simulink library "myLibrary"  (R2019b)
settings: Solver=VariableStepAuto  StartTime=0.0  StopTime=10.0  RelTol=1e-3
undefined symbols (not defined in the file or in its folder): batt_delay, Calculation, cap_1ph, cap_3ph, Complex, Current, Dynamic, EV, ev_charger, EV_ID, ev_num, gcbh, Iabc, Load, max_charge_1ph, max_charge_3ph, max_disch_1ph, max_disch_3ph, MV_LV_transf, myLibrary, phase, Phase, Phasor, rated_1ph, rated_3ph, Single, SoC_init, SPDL, sps_rtmsupport, Tr_capacity, Tstep, Vabc, Vnom, yes
libraries: powerlib x163, $bdroot x13, spsVIMeasurementModel x3, simulink x2, powerlib_meascontrol x1
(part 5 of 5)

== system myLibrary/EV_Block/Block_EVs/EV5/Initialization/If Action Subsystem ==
  Action Port : ActionPort
  Constant : Constant
  Out1 : Outport  VectorParamsAs1DForOutWhenUnconnected=off
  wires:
  Constant/1 -> Out1/1

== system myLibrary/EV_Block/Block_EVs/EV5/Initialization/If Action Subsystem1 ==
  Action Port : ActionPort
  Constant : Constant
  Out1 : Outport  VectorParamsAs1DForOutWhenUnconnected=off
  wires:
  Constant/1 -> Out1/1

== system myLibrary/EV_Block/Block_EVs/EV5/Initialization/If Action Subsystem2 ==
  Action Port : ActionPort
  Constant : Constant
  Out1 : Outport  VectorParamsAs1DForOutWhenUnconnected=off
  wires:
  Constant/1 -> Out1/1

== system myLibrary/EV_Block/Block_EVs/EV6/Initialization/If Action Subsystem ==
  Action Port : ActionPort
  Constant : Constant
  Out1 : Outport  VectorParamsAs1DForOutWhenUnconnected=off
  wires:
  Constant/1 -> Out1/1

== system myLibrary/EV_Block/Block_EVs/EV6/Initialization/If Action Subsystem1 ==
  Action Port : ActionPort
  Constant : Constant
  Out1 : Outport  VectorParamsAs1DForOutWhenUnconnected=off
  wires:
  Constant/1 -> Out1/1

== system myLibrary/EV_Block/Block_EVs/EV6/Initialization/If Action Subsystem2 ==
  Action Port : ActionPort
  Constant : Constant
  Out1 : Outport  VectorParamsAs1DForOutWhenUnconnected=off
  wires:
  Constant/1 -> Out1/1

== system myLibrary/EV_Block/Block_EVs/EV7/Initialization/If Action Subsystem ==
  Action Port : ActionPort
  Constant : Constant
  Out1 : Outport  VectorParamsAs1DForOutWhenUnconnected=off
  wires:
  Constant/1 -> Out1/1

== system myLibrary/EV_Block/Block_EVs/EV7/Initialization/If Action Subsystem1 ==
  Action Port : ActionPort
  Constant : Constant
  Out1 : Outport  VectorParamsAs1DForOutWhenUnconnected=off
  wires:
  Constant/1 -> Out1/1

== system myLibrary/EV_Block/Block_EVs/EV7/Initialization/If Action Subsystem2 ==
  Action Port : ActionPort
  Constant : Constant
  Out1 : Outport  VectorParamsAs1DForOutWhenUnconnected=off
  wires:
  Constant/1 -> Out1/1

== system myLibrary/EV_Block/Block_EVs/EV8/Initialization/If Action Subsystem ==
  Action Port : ActionPort
  Constant : Constant
  Out1 : Outport  VectorParamsAs1DForOutWhenUnconnected=off
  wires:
  Constant/1 -> Out1/1

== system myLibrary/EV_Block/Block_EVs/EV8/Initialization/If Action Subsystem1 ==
  Action Port : ActionPort
  Constant : Constant
  Out1 : Outport  VectorParamsAs1DForOutWhenUnconnected=off
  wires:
  Constant/1 -> Out1/1

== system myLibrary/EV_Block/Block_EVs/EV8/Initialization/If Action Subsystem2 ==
  Action Port : ActionPort
  Constant : Constant
  Out1 : Outport  VectorParamsAs1DForOutWhenUnconnected=off
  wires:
  Constant/1 -> Out1/1

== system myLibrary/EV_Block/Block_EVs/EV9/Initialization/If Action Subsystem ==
  Action Port : ActionPort
  Constant : Constant
  Out1 : Outport  VectorParamsAs1DForOutWhenUnconnected=off
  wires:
  Constant/1 -> Out1/1

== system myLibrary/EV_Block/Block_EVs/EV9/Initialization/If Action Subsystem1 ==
  Action Port : ActionPort
  Constant : Constant
  Out1 : Outport  VectorParamsAs1DForOutWhenUnconnected=off
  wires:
  Constant/1 -> Out1/1

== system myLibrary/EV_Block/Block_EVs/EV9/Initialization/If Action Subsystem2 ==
  Action Port : ActionPort
  Constant : Constant
  Out1 : Outport  VectorParamsAs1DForOutWhenUnconnected=off
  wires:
  Constant/1 -> Out1/1

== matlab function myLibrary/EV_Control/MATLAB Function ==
function [EV_cont_signals, k] = EV_Charging(EVsignals,P,Q,were_charging,ev_num, ev_charger, Tr_capacity)

EV_cont_signals=zeros(ev_num,1);
ev_charge=zeros(ev_num,1);
ev_time=zeros(ev_num,1);
list=zeros(ev_num,2);
list2=zeros(ev_num,2);
delay=4;
losses_per=8;
for i=1:ev_num
    ev_charge(i)=EVsignals(2*i-1);
    ev_time(i)=EVsignals(2*i);
end

%% available transformer capacity and EVs that can be charged

ev_charger=ev_charger*(1+losses_per/100);
Px=sqrt(Tr_capacity^2-Q^2);
DP=Px-P;
% consumption=consumption*(1+losses_per/100);
k=floor(DP/ev_charger); % how many cars the feeder can supply at this time step
c=sum(ev_charge); % how many cars want to charge at this time step
if k>0
if k>c
    for i=1:ev_num
        if ev_charge(i)==1
            EV_cont_signals(i)=1;
        end
    end
else
    j=1;
    m=1;
   for i=1:ev_num
       if were_charging(i)==1 && ev_charge(i)==1
           EV_cont_signals(i)=1;
           list(j,1)=i; % contains which cars were charging at t-1 and still want to charge at t
           list(j,2)=ev_time(i);
           j=j+1;
       elseif ev_charge(i)==1
           list2(m,1)=i;  % containts the cars that want to charge at t but were not charging at t-1
           list2(m,2)=ev_time(i);
           m=m+1;
       end
   end
   k2=nnz(list(:,1));
   k3=nnz(list2(:,1));
   k4=k-k2;
   
   if k2==k         
       if k3>0
           m=min(k3,k);
           for i=1:m
               [L1, IND1]=min(nonzeros(list(:,2)));
               [L2, IND2]=max(nonzeros(list2(:,2)));
               if (L2>=L1+delay) && (L1>1)
                  EV_cont_signals(list(IND1,1))=0;
                  EV_cont_signals(list2(IND2,1))=1;
                  
                  list(IND1:end-1,:)=list(IND1+1:end,:);
                  list(end,:)=0;
                  list2(IND2:end-1,:)=list2(IND2+1:end,:);
                  list2(end,:)=0;
                  
               else
                   break
               end
           end
       end
       
   elseif k>k2
       m=min(k3,k4);
       for i=1:m
           [L2, IND2]=max(nonzeros(list2(:,2)));
           EV_cont_signals(list2(IND2,1))=1;
           
           list2(IND2:end-1,:)=list2(IND2+1:end,:);
           list2(end,:)=0;
       end
       k3=nnz(list2(:,1));
       m=min(k3,k2);
       for i=1:m
               [L1, IND1]=min(nonzeros(list(:,2)));
               [L2, IND2]=max(nonzeros(list2(:,2)));
               if (L2>=L1+delay) && (L1>1)
                  EV_cont_signals(list(IND1,1))=0;
                  EV_cont_signals(list2(IND2,1))=1;
                  
                  list(IND1:end-1,:)=list(IND1+1:end,:);
                  list(end,:)=0;
                  list2(IND2:end-1,:)=list2(IND2+1:end,:);
                  list2(end,:)=0;
               else
                   break
               end
       end
       
   elseif k<k2
       for i=1:abs(k4)
           [L1, IND1]=min(nonzeros(list(:,2)));
           EV_cont_signals(list(IND1,1))=0;
           
           list(IND1:end-1,:)=list(IND1+1:end,:);
           list(end,:)=0;
       end
       k2=nnz(list(:,1));
       m=min(k3,k2);
       for i=1:m
               [L1, IND1]=min(nonzeros(list(:,2)));
               [L2, IND2]=max(nonzeros(list2(:,2)));
               if (L2>=L1+delay) && (L1>1)
                  EV_cont_signals(list(IND1,1))=0;
                  EV_cont_signals(list2(IND2,1))=1;
                  
                  list(IND1:end-1,:)=list(IND1+1:end,:);
                  list(end,:)=0;
                  list2(IND2:end-1,:)=list2(IND2+1:end,:);
                  list2(end,:)=0;
               else
                   break
               end
       end    
    end
 
end
end
